{attribute 'qualified_only'}
VAR_GLOBAL
	// Tc2_DALI
	{attribute 'TcContextName' := 'PlcCommunication'}
	stKL6821InDataTc2  		AT %I* 	: Tc2_DALI.ST_KL6821InData;	
	{attribute 'TcContextName' := 'PlcCommunication'}
    stKL6821OutDataTc2 		AT %Q* 	: Tc2_DALI.ST_KL6821OutData;
	stCommandBufferKL6821      		: Tc2_DALI.ST_DALIV2CommandBuffer;

	// Tc3_DALI
	{attribute 'TcContextName' := 'PlcCommunication'}
	stKL6821InDataTc3  		AT %I* 	: Tc3_DALI.ST_KL6821InData;	
	{attribute 'TcContextName' := 'PlcCommunication'}
    stKL6821OutDataTc3 		AT %Q* 	: Tc3_DALI.ST_KL6821OutData;
END_VAR
